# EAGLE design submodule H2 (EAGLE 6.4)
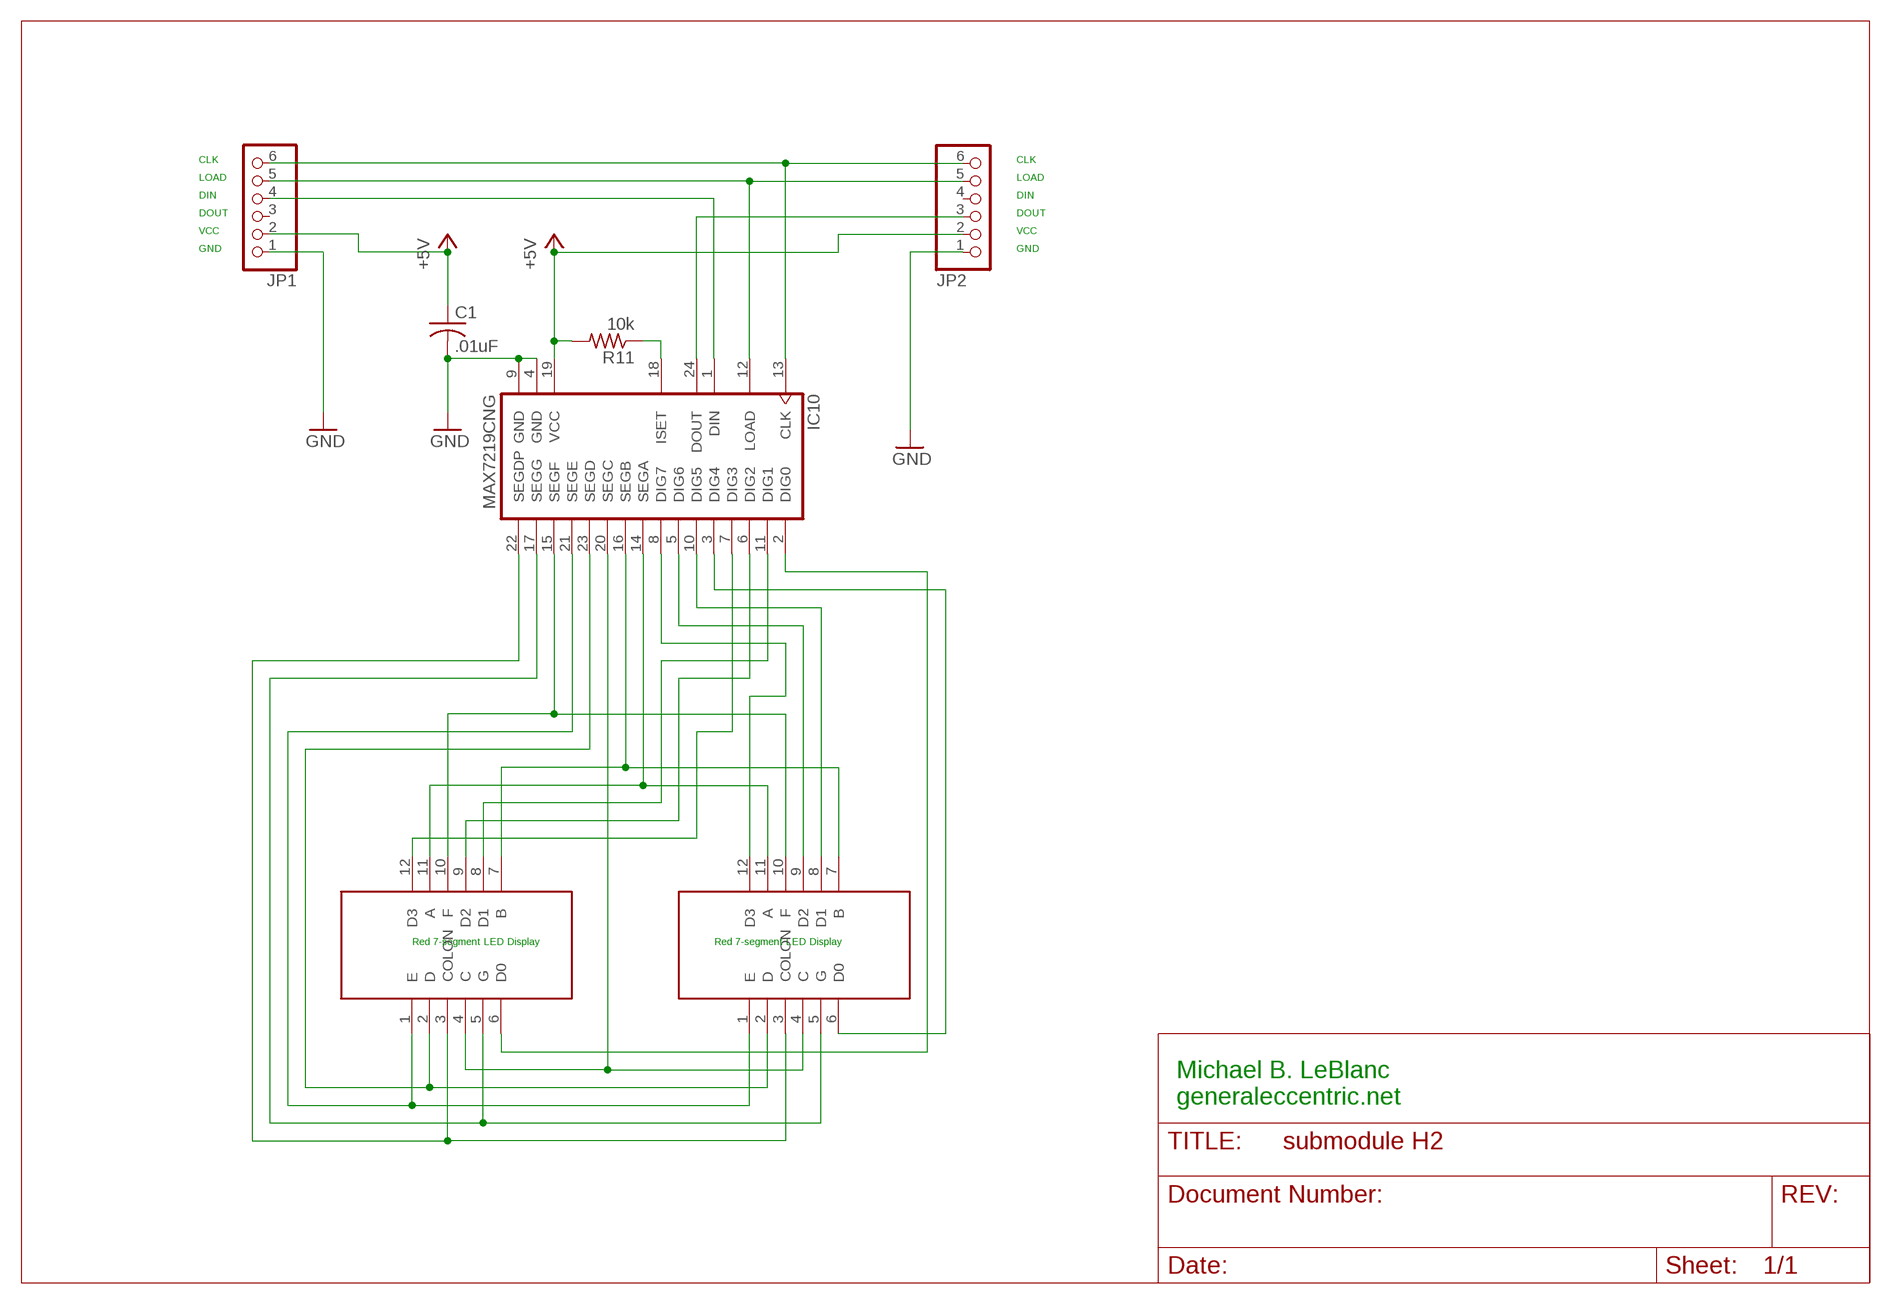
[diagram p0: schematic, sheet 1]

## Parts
C1  .01uF  C-US025-025X050  [C025-025X050]
IC10  MAX7219CNG  [DIL24-3]
JP1  PINHD-1X6  [1X06]
JP2  PINHD-1X6  [1X06]
R11  10k  R-US_0207/7  [0207/7]
U$1  CPS02841  [CPS02842]
U$2  CPS02841  [CPS02842]

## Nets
+5V: C1.1 IC10.19(VCC) JP1.2 JP2.2 R11.2
GND: C1.2 IC10.4(GND) IC10.9(GND) JP1.1 JP2.1
N$3: IC10.15(SEGF) U$1.10(F) U$2.10(F)
N$4: IC10.21(SEGE) U$1.1(E) U$2.1(E)
N$5: IC10.23(SEGD) U$1.2(D) U$2.2(D)
N$6: IC10.22(SEGDP) U$1.3(COLON) U$2.3(COLON)
N$7: IC10.20(SEGC) U$1.4(C) U$2.4(C)
N$8: IC10.16(SEGB) U$1.7(B) U$2.7(B)
N$9: IC10.14(SEGA) U$1.11(A) U$2.11(A)
N$10: IC10.2(DIG0) U$1.6(D0)
N$11: IC10.11(DIG1) U$1.8(D1)
N$12: IC10.6(DIG2) U$1.9(D2)
N$13: IC10.7(DIG3) U$1.12(D3)
N$14: IC10.3(DIG4) U$2.6(D0)
N$15: IC10.17(SEGG) U$1.5(G) U$2.5(G)
N$16: IC10.10(DIG5) U$2.8(D1)
N$17: IC10.5(DIG6) U$2.9(D2)
N$18: IC10.8(DIG7) U$2.12(D3)
N$21: IC10.24(DOUT) JP2.3
N$22: IC10.13(CLK) JP1.6 JP2.6
N$23: IC10.12(LOAD) JP1.5 JP2.5
N$24: IC10.1(DIN) JP1.4
N$25: IC10.18(ISET) R11.1
Unconnected: JP1.3 JP2.4

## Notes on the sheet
- CLK | CLK
- LOAD | LOAD
- DIN | DIN
- DOUT | DOUT
- VCC | VCC
- GND | GND
- Red 7-segment LED Display | Red 7-segment LED Display
- Michael B. LeBlanc
  generaleccentric.net

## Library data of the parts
C1 = adafruit:C-US: CAPACITOR, American symbol
IC10 = maxim:MAX7219CNG: LED DISPLAY DRIVER; MF: MAXIM; MPN: MAX7219CNG; OC_FARNELL: 1523914; OC_NEWARK: 34C4018
JP1 JP2 = adafruit:PINHD-1X6: PIN HEADER
R11 = adafruit:R-US_: RESISTOR, American symbol
U$1 U$2 = CPS02841:CPS02841: Four digit seven segment display.

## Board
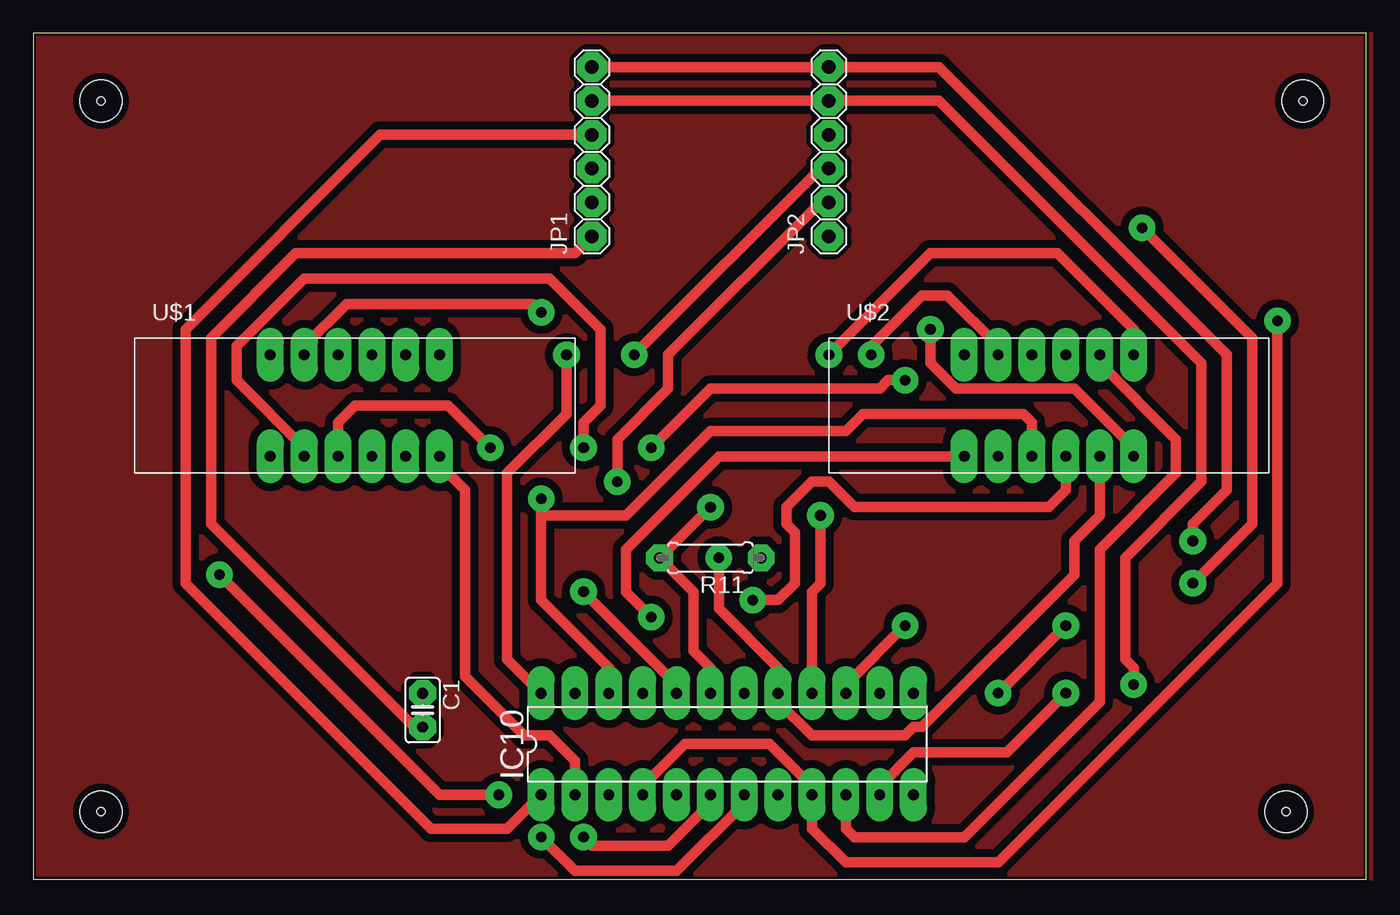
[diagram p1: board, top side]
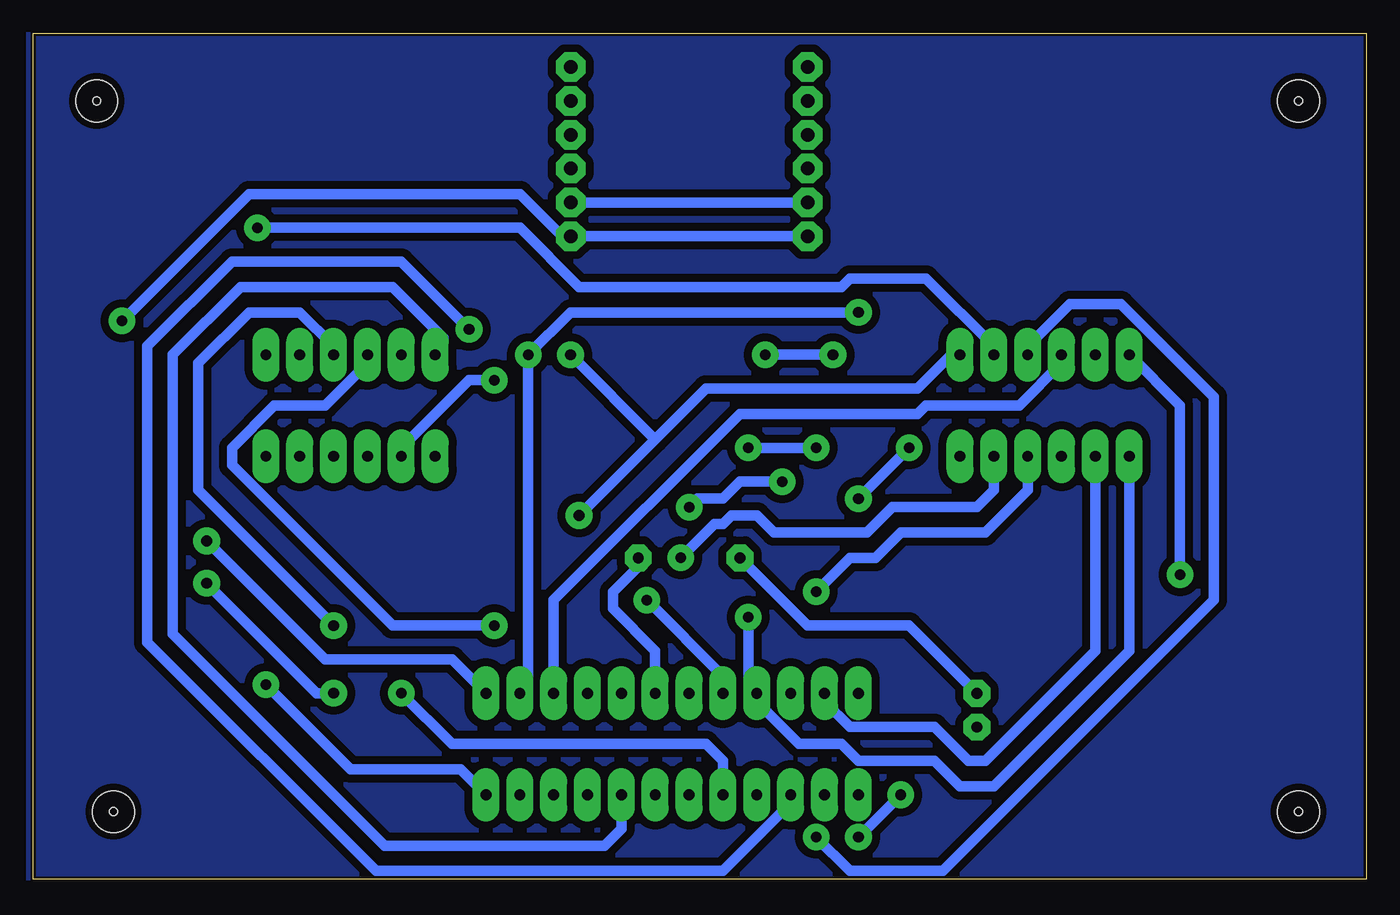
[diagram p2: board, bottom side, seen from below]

Size 100 x 63.49 mm. Coordinates in mm from the lower left corner, seen from the top.
Outline: 0,0 100,0 100,63.49 0,63.49 0,0
Copper layers (1*16): Top 0.035mm / dielectric 1.5mm / Bottom 0.035mm
Design rules: minimum track width 0.8mm, minimum drill 0.8mm, track to track 0.6mm, track to pad 0.6mm, pad to pad 0.45mm, via to via 0.8mm, smd to smd 8mil, copper to edge 8mil, drill to drill 8mil, minimum pad ring 0.6mm, minimum via ring 0.6mm, stop-mask expansion 0mil, vias tented up to drill 0mil, thermal gap 10mil
Holes 0.6 mm at 5.08,58.42 95.25,58.42 93.98,5.08 5.08,5.08
Holes 3.14 mm at 5.08,58.42 5.08,5.08 93.98,5.08 95.25,58.42

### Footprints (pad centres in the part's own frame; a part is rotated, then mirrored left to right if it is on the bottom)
C025-025X050 = drill 0.813 pad 1.676 octagon: 1 -1.27,0; 2 1.27,0
DIL24-3 = drill 0.813 long: 1 -13.97,-3.81; 2 -11.43,-3.81; 3 -8.89,-3.81; 4 -6.35,-3.81; 5 -3.81,-3.81; 6 -1.27,-3.81; 7 1.27,-3.81; 8 3.81,-3.81; 9 6.35,-3.81; 10 8.89,-3.81; 11 11.43,-3.81; 12 13.97,-3.81; 13 13.97,3.81; 14 11.43,3.81; 15 8.89,3.81; 16 6.35,3.81; 17 3.81,3.81; 18 1.27,3.81; 19 -1.27,3.81; 20 -3.81,3.81; 21 -6.35,3.81; 22 -8.89,3.81; 23 -11.43,3.81; 24 -13.97,3.81
1X06 = drill 1.016 octagon: 1 -6.35,0; 2 -3.81,0; 3 -1.27,0; 4 1.27,0; 5 3.81,0; 6 6.35,0
0207/7 = drill 0.813 octagon: 1 -3.81,0; 2 3.81,0
CPS02842 = drill 0.813 long: 1 -6.35,-3.81; 2 -3.81,-3.81; 3 -1.27,-3.81; 4 1.27,-3.81; 5 3.81,-3.81; 6 6.35,-3.81; 7 6.35,3.81; 8 3.81,3.81; 9 1.27,3.81; 10 -1.27,3.81; 11 -3.81,3.81; 12 -6.35,3.81

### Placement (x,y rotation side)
C1  29.21,12.7 270 top
IC10  52.07,10.16 0 top
JP1  41.91,54.61 90 top
JP2  59.69,54.61 90 top
R11  50.8,24.13 180 top
U$1  24.13,35.56 0 top
U$2  76.2,35.56 0 top

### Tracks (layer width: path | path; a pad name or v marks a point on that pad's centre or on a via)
+5V  (via drill 0.8)
  Top 0.8: 47.62,23.5 49.53,21.59 49.53,17.14 50.8,15.88 IC10.19 | JP2.2 59.05,50.8 47.62,39.37 47.62,36.83 43.81,33.02 v43.81,29.84 | v50.8,27.94 47.62,24.77 47.62,23.5 | 47.62,23.5 R11.2
  Bottom 0.8: JP2.2 JP1.2 | v43.81,29.84 46.99,29.84 48.26,28.57 50.16,28.57 v50.8,27.94 | C1.1 34.29,19.05 41.91,19.05 R11.2
GND  (via drill 0.8)
  Top 0.8: IC10.4 45.72,6.99 48.9,10.16 55.24,10.16 58.42,6.99 IC10.9 58.42,3.81 60.96,1.27 72.39,1.27 93.34,22.23 v93.34,41.91 | C1.2 28.57,11.43 13.34,26.67 13.34,40.64 19.68,46.99 40.64,46.99 JP1.1
  Bottom 0.8: JP1.1 JP2.1 60.33,48.26 63.5,51.44 83.82,51.44 v93.34,41.91
N$1
  pour Bottom: 0,63.5 100.33,63.5 100.33,0 0,0
N$2
  pour Top: 0,63.5 100.33,63.5 100.33,0 0,0
N$3  (via drill 0.8)
  Top 0.8: v65.41,19.05 60.96,14.61 IC10.15
  Bottom 0.8: U$1.10 22.86,38.73 26.04,35.56 33.02,35.56 33.66,34.92 46.99,34.92 60.96,20.95 IC10.15 | U$2.10 74.93,38.73 78.11,35.56 81.92,35.56 85.09,32.38 85.09,31.11 73.03,19.05 v65.41,19.05
N$4  (via drill 0.8)
  Top 0.8: U$2.1 51.44,31.75 44.45,24.77 44.45,21.59 v46.35,19.68
  Bottom 0.8: U$1.1 17.78,17.14 27.94,6.99 30.48,6.99 32.38,8.89 38.1,8.89 39.37,10.16 42.55,10.16 45.72,13.34 IC10.21 45.72,14.61 46.35,15.24 v46.35,19.68
N$5  (via drill 0.8)
  Top 0.8: v65.41,37.47 64.14,37.47 63.5,36.83 50.8,36.83 v46.35,32.38 | v41.27,32.38 41.27,34.29 42.55,35.56 42.55,41.27 38.73,45.09 20.32,45.09 15.24,40.01 15.24,37.47 20.32,32.38 U$1.2
  Bottom 0.8: IC10.23 40.64,13.34 38.73,11.43 32.38,11.43 29.84,8.89 28.57,8.89 20.32,17.14 U$1.2 | U$2.2 72.39,32.38 67.31,37.47 v65.41,37.47 | v41.27,32.38 v46.35,32.38
N$6  (via drill 0.8)
  Top 0.8: U$1.3 22.86,34.29 24.13,35.56 31.11,35.56 v34.29,32.38 | 38.1,27.3 38.1,20.95 43.18,15.88 IC10.22 | 38.1,27.3 v38.1,28.57 | U$2.3 74.93,34.29 74.3,34.92 62.23,34.92 60.96,33.66 50.8,33.66 44.45,27.3 38.1,27.3
  Bottom 0.8: v38.1,28.57 v34.29,32.38
N$7  (via drill 0.8)
  Top 0.8: v41.27,21.59 48.26,14.61 IC10.20 | U$2.4 77.47,29.21 76.2,27.94 61.59,27.94 59.69,29.84 58.42,29.84 56.52,27.94 56.52,26.67 57.15,26.04 57.15,22.23 55.88,20.95 v53.98,20.95
  Bottom 0.8: U$1.4 25.4,29.21 28.57,26.04 34.92,26.04 36.83,24.13 38.73,24.13 v41.27,21.59 | v53.98,20.95 48.26,15.24 IC10.20
N$8  (via drill 0.8)
  Top 0.8: IC10.16 58.42,21.59 59.05,22.23 v59.05,27.3 | U$2.7 82.55,41.27 76.83,46.99 67.31,46.99 v59.69,39.37
  Bottom 0.8: 53.34,33.02 49.53,36.83 33.66,36.83 31.11,39.37 U$1.7 | 53.34,33.02 v59.05,27.3 | 53.34,33.02 v59.69,39.37
N$9  (via drill 0.8)
  Top 0.8: U$1.11 20.32,40.01 23.5,43.18 37.47,43.18 v38.1,42.55 | U$2.11 72.39,40.01 68.58,43.81 66.67,43.81 62.87,40.01 v62.87,39.37
  Bottom 0.8: v38.1,42.55 59.69,42.55 v62.87,39.37 62.87,15.24 63.5,14.61 IC10.14
N$10
  Top 0.8: IC10.2 40.64,8.89 38.73,10.79 36.83,10.79 32.38,15.24 32.38,29.21 30.48,31.11 U$1.6
N$11  (via drill 0.8)
  Top 0.8: IC10.11 63.5,6.99 66.04,9.53 73.03,9.53 v77.47,13.97 | v87,22.23 91.44,26.67 91.44,40.64 v83.19,48.9
  Bottom 0.8: v77.47,13.97 78.74,13.97 v87,22.23 | v83.19,48.9 63.5,48.9 59.05,44.45 39.37,44.45 38.73,45.09 33.02,45.09 27.94,40.01 U$1.8
N$12  (via drill 0.8)
  Top 0.8: IC10.6 50.8,5.71 47.62,2.54 41.91,2.54 v41.27,3.17
  Bottom 0.8: v41.27,3.17 38.73,0.64 31.75,0.64 11.43,20.95 11.43,36.2 18.41,43.18 22.23,43.18 25.4,40.01 U$1.9
N$13  (via drill 0.8)
  Top 0.8: IC10.7 53.34,5.71 48.26,0.64 40.64,0.64 v38.1,3.17 | v34.92,6.35 30.48,6.35 v13.97,22.86
  Bottom 0.8: v34.92,6.35 v38.1,3.17 | v13.97,22.86 13.97,35.56 U$1.12
N$14  (via drill 0.8)
  Top 0.8: v67.31,41.27 67.31,38.73 69.22,36.83 78.11,36.83 82.55,32.38 U$2.6
  Bottom 0.8: IC10.3 43.18,5.71 48.26,0.64 74.3,0.64 91.44,17.78 91.44,40.01 85.09,46.35 72.39,46.35 v67.31,41.27
N$15  (via drill 0.8)
  Top 0.8: v51.44,24.13 51.44,20.32 55.88,15.88 IC10.17 55.88,13.34 58.42,10.79 65.41,10.79 66.04,11.43 66.67,11.43 78.11,22.86 78.11,25.4 80.01,27.3 U$2.5
  Bottom 0.8: U$1.5 27.94,29.21 29.21,27.94 35.56,27.94 37.47,26.04 44.45,26.04 45.72,27.3 47.62,27.3 48.26,26.67 48.9,26.67 v51.44,24.13
N$16
  Top 0.8: IC10.10 60.96,3.81 61.59,3.17 69.85,3.17 80.01,13.34 80.01,24.77 85.72,30.48 85.72,33.02 80.01,38.73 U$2.8
N$17  (via drill 0.8)
  Top 0.8: v77.47,19.05 v72.39,13.97
  Bottom 0.8: IC10.5 48.26,8.89 49.53,10.16 68.58,10.16 v72.39,13.97 | v77.47,19.05 87.63,29.21 87.63,38.73 83.82,42.55 80.01,42.55 77.47,40.01 U$2.9
N$18
  Bottom 0.8: IC10.8 55.88,3.81 57.15,2.54 73.66,2.54 89.53,18.41 89.53,39.37 84.45,44.45 73.03,44.45 69.22,40.64 69.85,40.01 U$2.12
N$21  (via drill 0.8)
  Top 0.8: IC10.24 35.56,16.51 35.56,30.48 40.01,34.92 v40.01,39.37 | v45.09,39.37 59.05,53.34 JP2.3
  Bottom 0.8: v45.09,39.37 v40.01,39.37
N$22  (via drill 0.8)
  Top 0.8: v87,25.4 87,26.67 89.53,29.21 89.53,39.37 67.94,60.96 JP2.6 JP1.6
  Bottom 0.8: IC10.13 68.58,16.51 78.11,16.51 v87,25.4
N$23  (via drill 0.8)
  Top 0.8: v82.55,14.61 82.55,15.88 81.92,16.51 81.92,24.13 87.63,29.84 87.63,38.73 67.94,58.42 JP2.5 JP1.5
  Bottom 0.8: IC10.12 67.94,8.26 76.2,8.26 v82.55,14.61
N$24
  Top 0.8: IC10.1 35.56,3.81 29.84,3.81 11.43,22.23 11.43,41.27 26.04,55.88 JP1.4
N$25
  Bottom 0.8: IC10.18 53.34,17.14 56.52,20.32 56.52,21.59 54.61,23.5 R11.1
(copper drawn outside any net)
  shapes: Bottom circle x4, Top circle x4

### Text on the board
tKeepout: Top
bKeepout: Bottom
